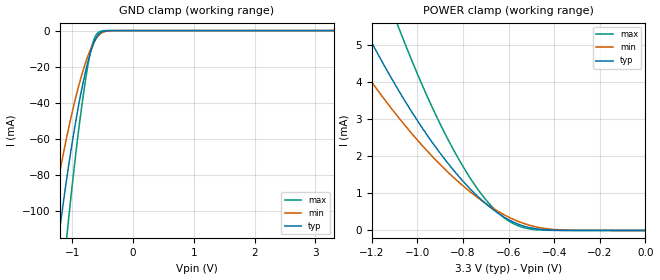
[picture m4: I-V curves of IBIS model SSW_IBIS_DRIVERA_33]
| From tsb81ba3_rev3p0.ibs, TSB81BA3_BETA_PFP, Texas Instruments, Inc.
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[Model]   SSW_IBIS_DRIVERA_33
Model_type  Input
Vinl=1.05
Vinh=2.34
| variable   typ   min   max
C_comp   4.06pF   3.33pF   5.79pF
[Temperature Range]   40   125   -40
| Ambient temperature   25   110   -40
[Voltage range]   3.3   3   3.6
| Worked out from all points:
|   GND clamp passes 1 mA (typ) near -0.53 V on its own axis
|   POWER clamp passes 1 mA (typ) near -0.75 V on its own axis
[GND Clamp]
| SSW_IBIS_DRIVERA_33
|   Voltage   I(typ)   I(min)   I(max)
-3.3V     -872mA     -653.5mA   -1.127A
-1.375V   -155.6mA   -110.7mA   -218.7mA
-1.205V   -109.5mA   -78.23mA   -154mA
-1.085V   -80.38mA   -57.91mA   -112.3mA
-905mV    -42.96mA   -31.92mA   -57.6mA
-770mV    -20.93mA   -16.56mA   -24.64mA
-720mV    -14.41mA   -11.97mA   -14.97mA
-670mV    -8.987mA   -8.11mA    -7.646mA
-615mV    -4.504mA   -4.792mA   -2.762mA
-560mV    -1.783mA   -2.49mA    -716.5uA
-280mV    -1.85uA    -13.46uA   -46.49nA
3.3V      4.137nA    3.673uA    3.789nA
[POWER Clamp]
| SSW_IBIS_DRIVERA_33
|   Voltage   I(typ)   I(min)   I(max)
-3.3V     43.87mA    33.08mA    62.52mA
-1.375V   7.208mA    5.576mA    10.7mA
-1.35V    6.881mA    5.336mA    10.21mA
-1.22V    5.279mA    4.156mA    7.779mA
-1.095V   3.894mA    3.131mA    5.658mA
-1.075V   3.687mA    2.978mA    5.34mA
-935mV    2.368mA    1.993mA    3.309mA
-805mV    1.358mA    1.226mA    1.77mA
-705mV    746uA      745.2uA    863.2uA
-620mV    358.9uA    422.9uA    341.9uA
-410mV    9.561uA    31.4uA     3.014uA
-48.03fV  4.137nA    21.05nA    4.157nA
